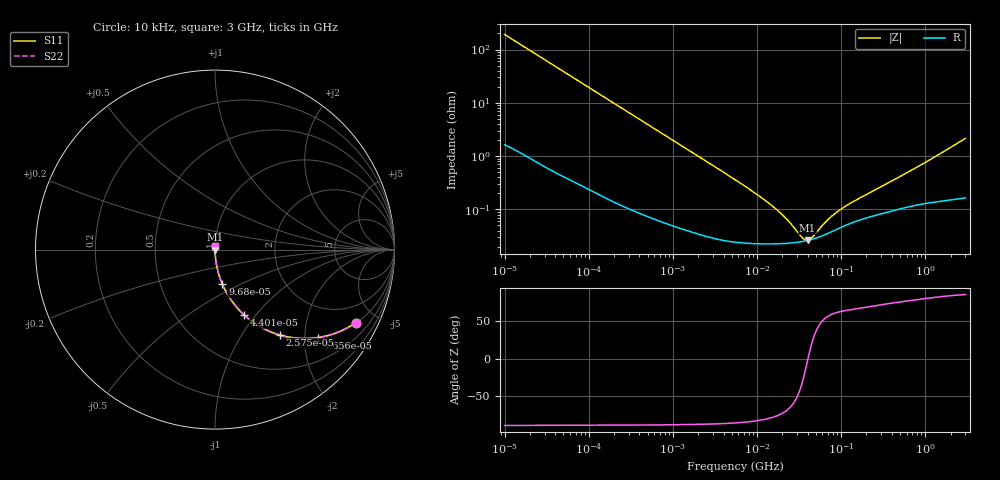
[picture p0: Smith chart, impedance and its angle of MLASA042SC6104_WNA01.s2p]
! MLASA042SC6104_WNA01  S-PARAMETER MODEL  ( Standard Model )
! Model Generated by TAIYO YUDEN Corporation (http://www.ty-top.com)
! Version 1.0
! TAIYO YUDEN Control No. 230906
! Copyright(c) 2023 TAIYO YUDEN CO.,LTD. All Rights Reserved.
! Product Description (link to TY-COMPAS)
! https://ds.yuden.co.jp/TYCOMPAS/or/detail?pn=MLASA042SC6104MWNA01&u=M
! Products Name : Multilayer Ceramic Capacitors
! Characteristics :
!  Capacitance : 0.1 [uF] , Rated Voltage : 4 [V] , TCC : X6S
!  Case Size : 0.4 x 0.2 / 0.016 x 0.008 [mm/inch] , Thickness : 0.2 / 0.008 [mm/inch]
!  (Conditions: Temperature = 25 [degC] , DC Bias Voltage = 0 [V])
! External Node Assignments :
!  1  o---| |---o  2
! GND o---------o GND
! Frequency Range : 10kHz  -  3GHz  [ 401 STEP ]
# MHZ S RI R 50
! Freq[MHz].  S11 Real  S11 Imag  S21 Real  S21 Imag  S12 Real  S12 Imag  S22 Real  S22 Imag
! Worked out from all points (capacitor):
!   401 points, 10 kHz to 3 GHz, reference 50 ohm
!   read as one part in series: C = 82.9 nF near 10.65 kHz
!   lowest |Z| = 26.1 mohm at 39.92 MHz (marker M1)
!   series resonance near 40.41 MHz, so ESL is about 190 pH
!   S11 on the Smith chart (normalised r, x): 10 kHz: 1.03, -3.83; 16.56 kHz: 1.02, -2.32; 25.75 kHz: 1.01, -1.50; 44.01 kHz: 1.01, -0.88; 96.8 kHz: 1.00, -0.40; 3 GHz: 1.00, +0.04
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0.01  0.7839 -0.4073  0.2161 0.4073  0.2161 0.4073  0.7839 -0.4073
0.016561  0.5733 -0.49  0.4267 0.49  0.4267 0.49  0.5733 -0.49
0.02575  0.3604 -0.4753  0.6396 0.4753  0.6396 0.4753  0.3604 -0.4753
0.044011  0.1643 -0.3654  0.8357 0.3654  0.8357 0.3654  0.1643 -0.3654
0.058452  0.1015 -0.2966  0.8985 0.2966  0.8985 0.2966  0.1015 -0.2966
0.082683  0.0546 -0.2214  0.9454 0.2214  0.9454 0.2214  0.0546 -0.2214
0.096801  0.0409 -0.1921  0.9591 0.1921  0.9591 0.1921  0.0409 -0.1921
0.226771  0.00859 -0.0854  0.9914 0.0854  0.9914 0.0854  0.00859 -0.0854
0.683653  0.00144 -0.0288  0.9986 0.0288  0.9986 0.0288  0.00144 -0.0288
5.477226  0.000255 -0.0036  0.9997 0.0036  0.9997 0.0036  0.000255 -0.0036
10.29003  0.000229 -0.00183  0.9998 0.00183  0.9998 0.00183  0.000229 -0.00183
15.99985  0.000226 -0.00106  0.9998 0.00106  0.9998 0.00106  0.000226 -0.00106
22.63272  0.000231 -0.000609  0.9998 0.000609  0.9998 0.000609  0.000231 -0.000609
34.09912  0.000248 -0.000168  0.9998 0.000168  0.9998 0.000168  0.000248 -0.000168
37.4819  0.000255 -7.4e-05  0.9997 7.4e-05  0.9997 7.4e-05  0.000255 -7.4e-05
39.92153  0.000261 -1.18e-05  0.9997 1.18e-05  0.9997 1.18e-05  0.000261 -1.18e-05
45.28751  0.000274 0.000112  0.9997 -0.000112  0.9997 -0.000112  0.000274 0.000112
66.11379  0.000341 0.000482  0.9997 -0.000482  0.9997 -0.000482  0.000341 0.000482
93.52181  0.000438 0.000833  0.9996 -0.000833  0.9996 -0.000833  0.000438 0.000833
140.9027  0.000576 0.00129  0.9994 -0.00129  0.9994 -0.00129  0.000576 0.00129
374.4521  0.000913 0.00308  0.9991 -0.00308  0.9991 -0.00308  0.000913 0.00308
3000  0.0021 0.0214  0.9979 -0.0214  0.9979 -0.0214  0.0021 0.0214
